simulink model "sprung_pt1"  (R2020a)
settings: Solver=ode45  StartTime=0.0  StopTime=10.0  RelTol=1e-3  EnableMultiTasking=on

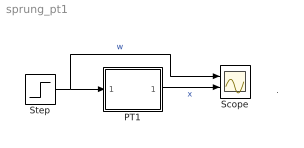
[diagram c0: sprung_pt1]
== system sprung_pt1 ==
  note: .
  PT1 : Subsystem  mask(PT1){T=2, Kp=5}
      mask prompts: T "Verzoegerungszeit"; Kp "Verstaerkung"
      mask help: Regelstrecke: einfaches Verzoegerungsglied vom PT1-Typ
  Scope : Scope  NumInputPorts=2
  Step : Step  SampleTime=0
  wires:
  Step/1 -> PT1/1(u), Scope/1  "w"
  PT1/1(x) -> Scope/2  "x"

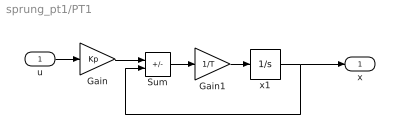
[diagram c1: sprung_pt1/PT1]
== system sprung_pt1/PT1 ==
  u : Inport
  Gain : Gain  Gain=Kp  SaturateOnIntegerOverflow=on
  Gain1 : Gain  Gain=1/T  SaturateOnIntegerOverflow=on
  Sum : Sum  Inputs=+-  SaturateOnIntegerOverflow=on
  x1 : Integrator
  x : Outport
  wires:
  Gain1/1 -> x1/1
  Sum/1 -> Gain1/1
  x1/1 -> Sum/2, x/1
  Gain/1 -> Sum/1
  u/1 -> Gain/1
